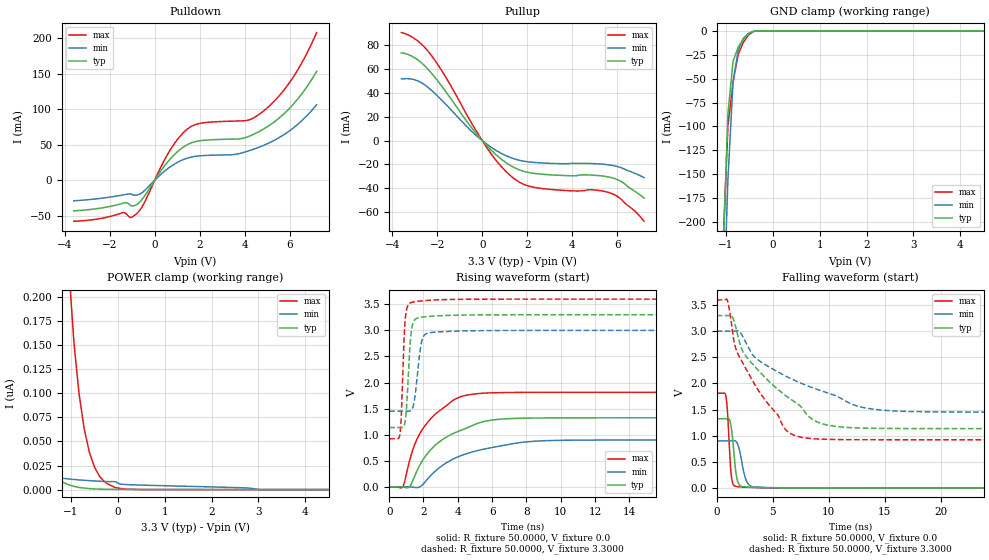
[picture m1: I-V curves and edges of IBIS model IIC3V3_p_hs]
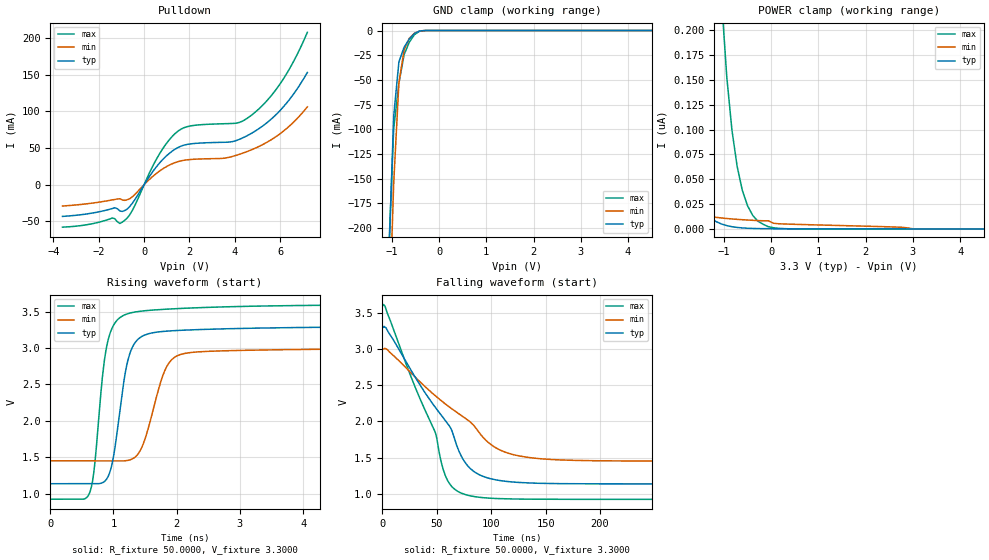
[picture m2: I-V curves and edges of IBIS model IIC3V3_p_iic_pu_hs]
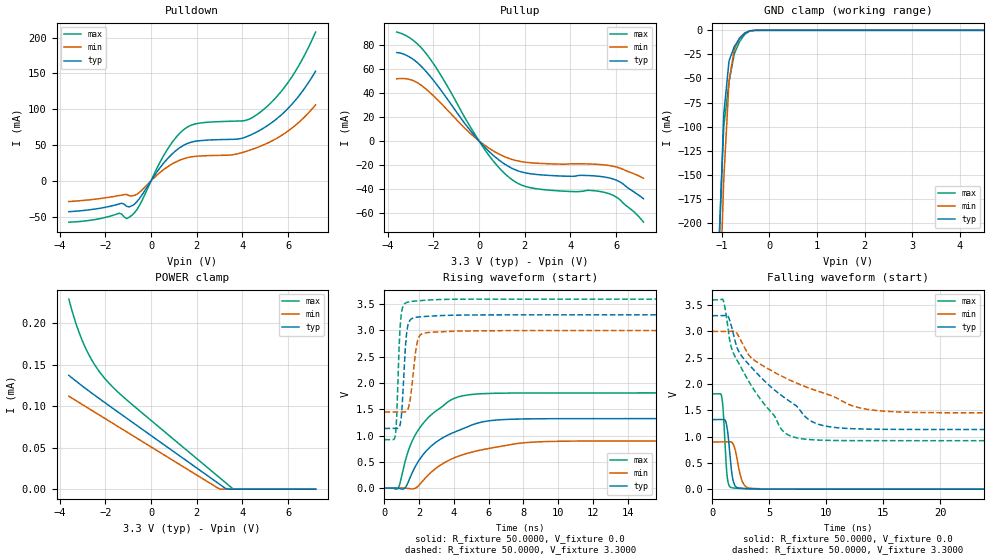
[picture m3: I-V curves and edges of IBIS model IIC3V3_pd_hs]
| IBIS file qfp64afe_3p3v.ibs generated by Viper version: 2020.12.17
[IBIS Ver]   5.0
[Comment Char]   |_char
[File Name]   qfp64afe_3p3v.ibs
[File Rev]   1.3
[Date]   Thu Dec 17 17:52:32 2020
[Source]   NXP Viper 2020.12.17
[Notes]
[Disclaimer] IMPORTANT NOTICE
  This information is provided on an AS IS basis and without warranty.
  IN NO EVENT SHALL NXP BE LIABLE FOR INCIDENTAL OR CONSEQUENTIAL
  DAMAGES ARISING FROM USE OF THIS INFORMATION. THIS DISCLAIMER OF
  WARRANTY EXTENDS TO THE USER OF THE INFORMATION, AND TO THEIR CUSTOMERS
  OR USERS OF PRODUCTS  AND IS IN LIEU OF ALL WARRANTIES WHETHER EXPRESS,
  IMPLIED, OR STATUTORY, INCLUDING IMPLIED WARRANTIES OF MERCHANTABILITY
  OR FITNESS FOR PARTICULAR PURPOSE.
  NXP does not represent or warrant that the information furnished
  hereunder is free of infringement of any third party patents,
  copyrights, trade secrets, or other intellectual property rights.
  NXP does not represent or warrant that the information is free of
  defect, or that it meets any particular standard, requirements or need
  of the user of the infomation or their customers.
  NXP reserves the right to change the information in this file
  without notice.
   http://www.nxp.com
[Copyright]   (C) Copyright NXP 2004 - 2020, All Rights Reserved.
|   qfp64Afe
[Component]   qfp64Afe
[Manufacturer]   NXP
[Package]
| variable   typ   min   max
R_pkg   0.18002   0.098036   0.22836
L_pkg   3.270e-09   2.478e-09   3.882e-09
C_pkg   4.877e-13   4.194e-13   6.388e-13
[Pin] signal_name   model_name   R_pin   L_pin   C_pin
1   P2_1   gpio   0.20176   3.768e-09 4.934e-13
2   OPAMP2_INN   NC   0.18655   3.432e-09 5.614e-13
3   P0_1   gpio   0.1882   3.425e-09 5.543e-13
4   P1_0   gpio   0.18167   3.391e-09 4.852e-13
5   ADC1IN1B   NC   0.17508   3.272e-09 4.734e-13
6   ADC1IN1A   NC   0.17211   3.184e-09 4.709e-13
7   P0_11   gpio   0.17322   3.095e-09 4.516e-13
8   VDDA   POWER   NA   NA   NA
9   VREF_OUT   NC   0.098933  2.478e-09 5.107e-13
10   VREFP   NC   0.098036  2.682e-09 4.989e-13
11   VREFN   NC   0.10339   2.593e-09 5.200e-13
12   VSSA   GND   NA   NA   NA
13   P0_16   gpio   0.18219   3.272e-09 4.683e-13
14   P0_10   gpio   0.18473   3.372e-09 4.943e-13
15   P0_15   gpio   0.1948   3.518e-09 5.647e-13
16   P0_31   gpio   0.21166   3.882e-09 5.047e-13
17   P0_8   gpio   0.19981   3.690e-09 4.818e-13
18   OPAMP0_INN   NC   0.18485   3.354e-09 5.404e-13
19   P0_27   gpio   0.1771   3.251e-09 5.158e-13
20   OPAMP1_INN   NC   0.17264   3.242e-09 4.518e-13
21   XTAL32M_N   NC   0.17308   3.207e-09 4.514e-13
22   XTAL32M_P   NC   0.17099   3.143e-09 4.435e-13
23   RESETN   gpio   0.17312   3.058e-09 4.290e-13
24   VDD_CORE   POWER   NA   NA   NA
25   P1_22   gpio   0.17347   2.976e-09 4.359e-13
26   P0_17   gpio   0.17222   3.063e-09 4.368e-13
27   P0_7   gpio   0.17974   2.960e-09 4.541e-13
28   VDDE_2   POWER   NA   NA   NA
29   VSS_MAIN_PWR   GND   NA   NA   NA
30   VSS_MAIN   GND   NA   NA   NA
31   LX   NC   0.12471   2.527e-09 6.388e-13
32   VDD_MAIN_PWR   NC   NA   NA   NA
33   XTAL32K_P   NC   0.20305   3.722e-09 4.831e-13
34   XTAL32K_N   NC   0.18797   3.388e-09 5.425e-13
35   VBAT   NC   0.17937   3.272e-09 4.763e-13
36   P0_0   gpio   0.17575   3.216e-09 4.542e-13
37   P0_9   gpio   0.17142   3.151e-09 4.522e-13
38   P0_18   gpio   0.17027   3.108e-09 4.408e-13
39   P1_13   gpio   0.17092   3.083e-09 4.194e-13
40   P1_1   gpio   0.17351   3.079e-09 4.367e-13
41   P0_26   gpio   0.17937   3.140e-09 4.480e-13
42   P1_2   gpio   0.18924   3.260e-09 4.417e-13
43   P1_3   gpio   0.20575   3.278e-09 4.623e-13
44   VDDE_4   POWER   NA   NA   NA
45   P0_24   gpio   0.18768   3.277e-09 4.591e-13
46   P0_13   iic   0.19613   3.445e-09 5.506e-13
47   P0_14   iic   0.20782   3.616e-09 5.657e-13
48   P0_20   gpio   0.21594   3.876e-09 4.850e-13
49   P0_21   gpio   0.20723   3.837e-09 4.904e-13
50   P0_22   gpio   0.1962   3.547e-09 5.661e-13
51   P0_25   gpio   0.18792   3.420e-09 5.062e-13
52   P0_2   gpio   0.18663   3.397e-09 4.750e-13
53   P1_15   gpio   0.17882   3.273e-09 4.700e-13
54   P0_19   gpio   0.17446   3.156e-09 4.633e-13
55   P0_3   gpio   0.17673   3.008e-09 4.457e-13
56   VDDE_4   POWER   NA   NA   NA
57   P0_4   gpio   0.17637   3.003e-09 4.457e-13
58   P1_16   gpio   0.17537   3.170e-09 4.476e-13
59   P0_6   gpio   0.17935   3.248e-09 4.687e-13
60   P0_5   gpio   0.18758   3.378e-09 4.757e-13
61   P0_29   gpio   0.19171   3.430e-09 4.834e-13
62   P1_11   gpio   0.20582   3.539e-09 5.647e-13
63   P0_30   gpio   0.22836   3.428e-09 5.818e-13
64   VDDE_4   POWER   NA   NA   NA
65   VSS   GND   NA   NA   NA
[Pin Mapping]   pulldown_ref   pullup_ref
1   VSS   VDDA
2   NC   NC
3   VSS   VDDA
4   VSS   VDDA
5   NC   NC
6   NC   NC
7   VSS   VDDA
8   NC   VDDA
9   NC   NC
10   NC   NC
11   NC   NC
12   VSSA   NC
13   VSS   VDDA
14   VSS   VDDA
15   VSS   VDDA
16   VSS   VDDA
17   VSS   VDDA
18   NC   NC
19   VSS   VDDA
20   NC   NC
21   NC   NC
22   NC   NC
23   VSS   VDDE_2
24   NC   VDD_CORE
25   VSS   VDDE_2
26   VSS   VDDE_2
27   VSS   VDDE_2
28   NC   VDDE_2
29   VSS_MAIN_PWR   NC
30   VSS_MAIN   NC
31   NC   NC
32   NC   NC
33   NC   NC
34   NC   NC
35   NC   NC
36   VSS   VDDE_4
37   VSS   VDDE_4
38   VSS   VDDE_4
39   VSS   VDDE_4
40   VSS   VDDE_4
41   VSS   VDDE_4
42   VSS   VDDE_4
43   VSS   VDDE_4
44   NC   VDDE_4
45   VSS   VDDE_4
46   VSS   VDDE_4
47   VSS   VDDE_4
48   VSS   VDDE_4
49   VSS   VDDE_4
50   VSS   VDDE_4
51   VSS   VDDE_4
52   VSS   VDDE_4
53   VSS   VDDE_4
54   VSS   VDDE_4
55   VSS   VDDE_4
56   NC   VDDE_4
57   VSS   VDDE_4
58   VSS   VDDE_4
59   VSS   VDDE_4
60   VSS   VDDE_4
61   VSS   VDDE_4
62   VSS   VDDE_4
63   VSS   VDDE_4
64   NC   VDDE_4
65   VSS   NC
|*   Model Selector   *
[Model Selector] gpio
MFIO3V3_pd_hs   EPUN=1 EPD=1 EHS=1
MFIO3V3_pd_ls   EPUN=1 EPD=1 EHS=0
MFIO3V3_pu_hs   EPUN=0 EPD=0 EHS=1
MFIO3V3_pu_ls   EPUN=0 EPD=0 EHS=0
MFIO3V3_p_hs   EPUN=1 EPD=0 EHS=1
MFIO3V3_p_ls   EPUN=1 EPD=0 EHS=0
MFIO3V3_r_hs   EPUN=0 EPD=1 EHS=1
MFIO3V3_r_ls   EPUN=0 EPD=1 EHS=0
[Model Selector] iic
IIC3V3_pd_hs   EGP=1 EPUN=1 EPD=1 EHS=1
IIC3V3_pd_ls   EGP=1 EPUN=1 EPD=1 EHS=0
IIC3V3_p_hs   EGP=1 EPUN=1 EPD=0 EHS=1
IIC3V3_p_ls   EGP=1 EPUN=1 EPD=0 EHS=0
IIC3V3_pu_hs   EGP=1 EPUN=0 EPD=0 EHS=1
IIC3V3_pu_ls   EGP=1 EPUN=0 EPD=0 EHS=0
IIC3V3_r_hs   EGP=1 EPUN=0 EPD=1 EHS=1
IIC3V3_r_ls   EGP=1 EPUN=0 EPD=1 EHS=0
IIC3V3_pd_iic_hs   EGP=0 ECS=0 EPUN=1 EPD=1
IIC3V3_p_iic_hs   EGP=0 ECS=0 EPUN=1 EPD=0
IIC3V3_pu_iic_hs   EGP=0 ECS=0 EPUN=0 EPD=0
IIC3V3_r_iic_hs   EGP=0 ECS=0 EPUN=0 EPD=1
IIC3V3_pd_iic_pu_hs   EGP=0 ECS=1 EPUN=1 EPD=1 SSEL=1
IIC3V3_p_iic_pu_hs   EGP=0 ECS=1 EPUN=1 EPD=0 SSEL=1
IIC3V3_pu_iic_pu_hs   EGP=0 ECS=1 EPUN=0 EPD=0 SSEL=1
IIC3V3_r_iic_pu_hs   EGP=0 ECS=1 EPUN=0 EPD=1 SSEL=1
| End [Component] qfp64Afe
| Models and submodels in the file (24): IIC3V3_p_hs (I/O), IIC3V3_p_iic_hs (I/O_open_drain), IIC3V3_p_iic_pu_hs (I/O_open_drain), IIC3V3_p_ls (I/O), IIC3V3_pd_hs (I/O), IIC3V3_pd_iic_hs (I/O_open_drain), IIC3V3_pd_iic_pu_hs (I/O_open_drain), IIC3V3_pd_ls (I/O), IIC3V3_pu_hs (I/O), IIC3V3_pu_iic_hs (I/O_open_drain), IIC3V3_pu_iic_pu_hs (I/O_open_drain), IIC3V3_pu_ls (I/O), IIC3V3_r_hs (I/O), IIC3V3_r_iic_hs (I/O_open_drain), IIC3V3_r_iic_pu_hs (I/O_open_drain), IIC3V3_r_ls (I/O), MFIO3V3_p_hs (I/O), MFIO3V3_p_ls (I/O), MFIO3V3_pd_hs (I/O), MFIO3V3_pd_ls (I/O), MFIO3V3_pu_hs (I/O), MFIO3V3_pu_ls (I/O), MFIO3V3_r_hs (I/O), MFIO3V3_r_ls (I/O)
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[Model] IIC3V3_p_hs
|   Model IIC3V3_p_hs
| This model was characterised for following simulation conditions:
| External (pad) voltage:
|   - Typ: 3.3V,   - Min: 3.0V,   - Max: 3.6V
| Library cells for typ/min/max conditions are connected as defined below:
|  IO - External Pad
|  A - Core Input
|  EN - Output Buffer Enable
|  BOOST - vdde
|  EGP - vdd
|  EHS - vdd
|  ENZI - vdd
|  EPD - gnd
|  EPUN - vdd
|  ZI - NC
|  ZIF - NC
|  gnd - gnd
|  gnde - gnde
|  vdd - vdd
|  vdde - vdde
| All other pins connected to ground
Model_type I/O
Polarity   Non-Inverting
Enable   Active-Low
Vinl =   0.9900V
Vinh =   2.3100V
Vmeas =  1.6500V
Cref =   0.0F
Rref =   1.0000k
Vref =   0.0V
C_comp   3.6227pF   3.4779pF   3.7656pF
|C_comp_pullup   0.9287pF   0.9115pF   0.9356pF
|C_comp_pulldown   2.3426pF   2.4945pF   2.1982pF
[Model Spec]
| variable   typ   min   max
Vinh   0.9900V   0.9000V   1.0800V
Vinl   2.3100V   2.1000V   2.5200V
Vmeas   1.6500V   1.5000V   1.8000V
[Temperature Range]   25.0000   0.1250k   -40.0000
[Voltage Range]   3.3000V   3.0000V   3.6000V
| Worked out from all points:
|   slope of the pulldown table from 0 to 0.495 V, typ, clamps not added: 22 ohm
|   slope of the pullup table from 0 to 0.495 V, typ, clamps not added: 50.2 ohm
|   GND clamp passes 1 mA (typ) near -0.43 V on its own axis
|   rising waveform, R_fixture 50.0000, V_fixture 0.0: 20-80 % time 2.42ns typ, 3.15ns min, 1.81ns max; typ from 0 V to 1.32 V
|   rising waveform, R_fixture 50.0000, V_fixture 3.3000: 20-80 % time 230ps typ, 322ps min, 186ps max; typ from 1.14 V to 3.3 V
|   falling waveform, R_fixture 50.0000, V_fixture 0.0: 20-80 % time 371ps typ, 535ps min, 282ps max; typ from 1.32 V to 0 V
|   falling waveform, R_fixture 50.0000, V_fixture 3.3000: 20-80 % time 5.52ns typ, 7.85ns min, 3.84ns max; typ from 3.3 V to 1.14 V
[Pulldown]
|Voltage   I(typ)   I(min)   I(max)
-3.6V     -43.22mA   -29.09mA   -57.9mA
-1.29V    -31.46mA   -20.15mA   -46.47mA
-1.07V    -35.79mA   -19.19mA   -52.9mA
-850mV    -35.14mA   -21.36mA   -48.43mA
-520mV    -25.35mA   -16.52mA   -35.11mA
580mV     25.81mA    16.3mA     36.8mA
1.24V     45.79mA    28.53mA    65.82mA
1.9V      54.89mA    33.9mA     79.08mA
4.1V      60.56mA    40.39mA    84.05mA
4.76V     70.46mA    47.89mA    95.34mA
6.08V     103.9mA    71.43mA    141.2mA
7.2V      153mA      106.1mA    207.7mA
[Pullup]
|Voltage   I(typ)   I(min)   I(max)
-3.6V     73.7mA     51.87mA    90.79mA
-2.92V    68.56mA    50.58mA    84.45mA
-2.26V    56.64mA    42.24mA    71.49mA
-1.6V     40.55mA    30.05mA    52.55mA
160mV     -3.402mA   -2.371mA   -4.704mA
820mV     -15.2mA    -10.46mA   -21.22mA
1.37V     -22.16mA   -15.02mA   -31.28mA
1.81V     -25.65mA   -17.18mA   -36.45mA
2.47V     -27.92mA   -18.56mA   -39.79mA
5.66V     -30.76mA   -20.47mA   -43.83mA
6.1V      -33.55mA   -22.29mA   -48.04mA
7.2V      -48.27mA   -31.2mA    -67.82mA
[GND_clamp]
|Voltage   I(typ)   I(min)   I(max)
-3.6V     -5.602A    -5.487A    -5.717A
-1.07V    -242mA     -316.8mA   -230.5mA
-960mV    -86.75mA   -154.7mA   -99.48mA
-850mV    -31.81mA   -53.08mA   -53.5mA
-740mV    -16.96mA   -19.87mA   -24.43mA
-630mV    -8.589mA   -7.919mA   -11.88mA
-520mV    -2.996mA   -2.727mA   -4.187mA
-410mV    -432.5uA   -495.8uA   -580.8uA
7.2V      0A         0A         0A
[POWER_clamp]
|Voltage   I(typ)   I(min)   I(max)
-3.6V     2.12uA     118.8nA    63.41uA
-3.03V    844.5nA    61.84nA    27.62uA
-2.37V    225.8nA    29.91nA    8.403uA
-2.04V    102.5nA    21.72nA    4.105uA
-1.82V    57.11nA    17.98nA    2.406uA
-1.49V    21.61nA    14.11nA    975.4nA
-1.05V    4.967nA    11.05nA    231.3nA
-830mV    2.261nA    10.06nA    99.54nA
-720mV    1.525nA    9.658nA    63.01nA
-500mV    718.9pA    8.985nA    23.37nA
-170mV    294.4pA    8.237nA    4.755nA
7.2V      0A         0A         0A
[Ramp]
| variable   typ   min   max
dV/dt_r  0.7941/2.4211n   0.5390/3.1525n   1.0875/1.8120n
dV/dt_f  1.2989/5.5187n   0.9297/7.8507n   1.6070/3.8381n
R_load = 50.0000
[Rising Waveform]
R_fixture= 50.0000
V_fixture= 0.0
V_fixture_min= 0.0
V_fixture_max= 0.0
|time   V(typ)   V(min)   V(max)
0s        2.243nV    52.63nV    27.54nV
783.4ps   -2.546mV   48.23uV    -3.663mV
1.2ns     6.371mV    -1.183mV   516.9mV
1.762ns   400.2mV    -5.572mV   1.005V
2.604ns   772.3mV    274.8mV    1.368V
3.633ns   1.006V     515.9mV    1.636V
5.446ns   1.245V     716.8mV    1.794V
7.589ns   1.314V     845.6mV    1.81V
17.45ns   1.323V     898mV      1.812V
1us       1.323V     898.3mV    1.813V
[Rising Waveform]
R_fixture= 50.0000
V_fixture= 3.3000
V_fixture_min= 3.0000
V_fixture_max= 3.6000
|time   V(typ)   V(min)   V(max)
0s        1.135V     1.45V      921.7mV
627.3ps   1.135V     1.45V      1.012V
700.7ps   1.134V     1.451V     1.326V
903.6ps   1.208V     1.45V      3.068V
1.101ns   2.057V     1.448V     3.484V
1.223ns   2.763V     1.454V     3.525V
1.356ns   3.105V     1.506V     3.542V
2.023ns   3.26V      2.9V       3.57V
4.301ns   3.294V     2.99V      3.597V
1us       3.3V       3V         3.6V
[Falling Waveform]
R_fixture= 50.0000
V_fixture= 0.0
V_fixture_min= 0.0
V_fixture_max= 0.0
|time   V(typ)   V(min)   V(max)
0s        1.323V     898.3mV    1.813V
822ps     1.323V     898.3mV    1.758V
972.4ps   1.326V     898.3mV    1.431V
1.252ns   1.222V     898.1mV    350.6mV
1.476ns   816.9mV    900.3mV    64.93mV
1.726ns   277.3mV    889.4mV    27.64mV
2.019ns   57.27mV    737.3mV    19.74mV
2.754ns   14.85mV    95.71mV    10.98mV
4.273ns   3.379mV    7.479mV    1.748mV
1us       13.95nV    73.04nV    34.74nV
[Falling Waveform]
R_fixture= 50.0000
V_fixture= 3.3000
V_fixture_min= 3.0000
V_fixture_max= 3.6000
|time   V(typ)   V(min)   V(max)
0s        3.3V       3V         3.6V
933.7ps   3.299V     3V         3.603V
1.389ns   3.287V     2.999V     3.037V
1.891ns   2.917V     3.01V      2.567V
2.697ns   2.498V     2.747V     2.246V
6.123ns   1.774V     2.146V     1.125V
10.95ns   1.17V      1.732V     925.1mV
14.46ns   1.14V      1.495V     922mV
24.74ns   1.135V     1.451V     921.7mV
1us       1.135V     1.45V      921.7mV
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[Model] IIC3V3_p_iic_pu_hs
|   Model IIC3V3_p_iic_pu_hs
| This model was characterised for following simulation conditions:
| External (pad) voltage:
|   - Typ: 3.3V,   - Min: 3.0V,   - Max: 3.6V
| Library cells for typ/min/max conditions are connected as defined below:
|  IO - External Pad
|  A - Core Input
|  EN - Output Buffer Enable
|  BOOST - vdde
|  ECS - vdd
|  EGP - gnd
|  ENZI - vdd
|  EPD - gnd
|  EPUN - vdd
|  SSEL - vdd
|  ZI - NC
|  ZIF - NC
|  gnd - gnd
|  gnde - gnde
|  vdd - vdd
|  vdde - vdde
| All other pins connected to ground
Model_type I/O_open_drain
Polarity   Non-Inverting
Enable   Active-Low
Vinl =   0.9900V
Vinh =   2.3100V
Vmeas =  1.6500V
Cref =   0.0F
Rref =   1.0000k
Vref =   3.3000V
C_comp   3.6227pF   3.4779pF   3.7656pF
|C_comp_pullup   0.9287pF   0.9114pF   0.9356pF
|C_comp_pulldown   2.3426pF   2.4946pF   2.1982pF
[Model Spec]
| variable   typ   min   max
Vinh   0.9900V   0.9000V   1.0800V
Vinl   2.3100V   2.1000V   2.5200V
Vmeas   1.6500V   1.5000V   1.8000V
Vref   3.3000V   3.0000V   3.6000V
Cref   0.0F   0.0F   0.0F
Rref   1.0000k   1.0000k   1.0000k
[Temperature Range]   25.0000   0.1250k   -40.0000
[Voltage Range]   3.3000V   3.0000V   3.6000V
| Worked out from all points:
|   slope of the pulldown table from 0 to 0.495 V, typ, clamps not added: 22 ohm
|   GND clamp passes 1 mA (typ) near -0.43 V on its own axis
|   rising waveform, R_fixture 50.0000, V_fixture 3.3000: 20-80 % time 227ps typ, 309ps min, 192ps max; typ from 1.14 V to 3.3 V
|   falling waveform, R_fixture 50.0000, V_fixture 3.3000: 20-80 % time 50.8ns typ, 68.7ns min, 38.5ns max; typ from 3.3 V to 1.14 V
[Pulldown]
|Voltage   I(typ)   I(min)   I(max)
-3.6V     -43.22mA   -29.09mA   -57.9mA
-1.29V    -31.46mA   -20.15mA   -46.47mA
-1.07V    -35.79mA   -19.19mA   -52.9mA
-850mV    -35.14mA   -21.36mA   -48.43mA
-520mV    -25.35mA   -16.52mA   -35.11mA
580mV     25.81mA    16.3mA     36.8mA
1.24V     45.79mA    28.53mA    65.82mA
1.9V      54.89mA    33.9mA     79.08mA
4.1V      60.56mA    40.39mA    84.05mA
4.76V     70.46mA    47.89mA    95.34mA
6.08V     103.9mA    71.43mA    141.2mA
7.2V      153mA      106.1mA    207.7mA
[GND_clamp]
|Voltage   I(typ)   I(min)   I(max)
-3.6V     -5.602A    -5.487A    -5.717A
-1.07V    -242mA     -316.8mA   -230.5mA
-960mV    -86.75mA   -154.7mA   -99.48mA
-850mV    -31.81mA   -53.08mA   -53.5mA
-740mV    -16.96mA   -19.87mA   -24.43mA
-630mV    -8.589mA   -7.919mA   -11.88mA
-520mV    -2.996mA   -2.727mA   -4.187mA
-410mV    -432.5uA   -495.8uA   -580.8uA
7.2V      0A         0A         0A
[POWER_clamp]
|Voltage   I(typ)   I(min)   I(max)
-3.6V     2.12uA     118.8nA    63.41uA
-3.03V    844.5nA    61.84nA    27.62uA
-2.37V    225.8nA    29.91nA    8.403uA
-2.04V    102.5nA    21.72nA    4.105uA
-1.82V    57.11nA    17.98nA    2.406uA
-1.49V    21.61nA    14.11nA    975.4nA
-1.05V    4.967nA    11.05nA    231.3nA
-830mV    2.261nA    10.06nA    99.54nA
-720mV    1.525nA    9.658nA    63.01nA
-500mV    718.9pA    8.985nA    23.37nA
-170mV    294.4pA    8.237nA    4.755nA
7.2V      0A         0A         0A
[Ramp]
| variable   typ   min   max
dV/dt_r  1.2989/0.2271n   0.9297/0.3090n   1.6070/0.1925n
dV/dt_f  1.2989/50.7796n   0.9297/68.6526n   1.6070/38.5019n
R_load = 50.0000
[Rising Waveform]
R_fixture= 50.0000
V_fixture= 3.3000
V_fixture_min= 3.0000
V_fixture_max= 3.6000
|time   V(typ)   V(min)   V(max)
0s        1.135V     1.45V      921.7mV
623.4ps   1.135V     1.45V      1.013V
886ps     1.193V     1.45V      2.995V
994ps     1.479V     1.45V      3.305V
1.153ns   2.48V      1.449V     3.448V
1.388ns   3.122V     1.544V     3.503V
1.807ns   3.231V     2.682V     3.534V
2.03ns    3.244V     2.903V     3.544V
5.603ns   3.294V     2.992V     3.595V
1us       3.3V       3V         3.6V
[Falling Waveform]
R_fixture= 50.0000
V_fixture= 3.3000
V_fixture_min= 3.0000
V_fixture_max= 3.6000
|time   V(typ)   V(min)   V(max)
0s        3.3V       3V         3.6V
2.46ns    3.303V     3.01V      3.593V
48.38ns   2.199V     2.358V     1.857V
54.58ns   2.076V     2.28V      1.407V
59.71ns   1.976V     2.22V      1.188V
72.76ns   1.512V     2.08V      1.006V
83.18ns   1.317V     1.957V     962.6mV
112.4ns   1.172V     1.577V     928.9mV
163.4ns   1.139V     1.467V     922.1mV
1us       1.135V     1.45V      921.7mV
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[Model] IIC3V3_pd_hs
|   Model IIC3V3_pd_hs
| This model was characterised for following simulation conditions:
| External (pad) voltage:
|   - Typ: 3.3V,   - Min: 3.0V,   - Max: 3.6V
| Library cells for typ/min/max conditions are connected as defined below:
|  IO - External Pad
|  A - Core Input
|  EN - Output Buffer Enable
|  BOOST - vdde
|  EGP - vdd
|  EHS - vdd
|  ENZI - vdd
|  EPD - vdd
|  EPUN - vdd
|  ZI - NC
|  ZIF - NC
|  gnd - gnd
|  gnde - gnde
|  vdd - vdd
|  vdde - vdde
| All other pins connected to ground
Model_type I/O
Polarity   Non-Inverting
Enable   Active-Low
Vinl =   0.9900V
Vinh =   2.3100V
Vmeas =  1.6500V
Cref =   0.0F
Rref =   1.0000k
Vref =   0.0V
C_comp   3.5907pF   3.4406pF   3.7387pF
|C_comp_pullup   0.9138pF   0.9000pF   0.9174pF
|C_comp_pulldown   2.3267pF   2.4802pF   2.1806pF
[Model Spec]
| variable   typ   min   max
Vinh   0.9900V   0.9000V   1.0800V
Vinl   2.3100V   2.1000V   2.5200V
Vmeas   1.6500V   1.5000V   1.8000V
[Temperature Range]   25.0000   0.1250k   -40.0000
[Voltage Range]   3.3000V   3.0000V   3.6000V
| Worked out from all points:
|   slope of the pulldown table from 0 to 0.495 V, typ, clamps not added: 22 ohm
|   slope of the pullup table from 0 to 0.495 V, typ, clamps not added: 50.2 ohm
|   GND clamp passes 1 mA (typ) near -0.43 V on its own axis
|   rising waveform, R_fixture 50.0000, V_fixture 0.0: 20-80 % time 2.41ns typ, 3.15ns min, 1.81ns max; typ from 0 V to 1.32 V
|   rising waveform, R_fixture 50.0000, V_fixture 3.3000: 20-80 % time 230ps typ, 322ps min, 186ps max; typ from 1.14 V to 3.3 V
|   falling waveform, R_fixture 50.0000, V_fixture 0.0: 20-80 % time 371ps typ, 533ps min, 281ps max; typ from 1.32 V to 0 V
|   falling waveform, R_fixture 50.0000, V_fixture 3.3000: 20-80 % time 5.51ns typ, 7.83ns min, 3.82ns max; typ from 3.3 V to 1.14 V
[Pulldown]
|Voltage   I(typ)   I(min)   I(max)
-3.6V     -43.22mA   -29.09mA   -57.9mA
-1.29V    -31.46mA   -20.15mA   -46.47mA
-1.07V    -35.79mA   -19.19mA   -52.9mA
-850mV    -35.14mA   -21.36mA   -48.43mA
-520mV    -25.35mA   -16.52mA   -35.11mA
580mV     25.81mA    16.3mA     36.8mA
1.24V     45.79mA    28.53mA    65.82mA
1.9V      54.89mA    33.9mA     79.08mA
4.1V      60.55mA    40.38mA    84.05mA
4.76V     70.44mA    47.87mA    95.32mA
6.08V     103.9mA    71.39mA    141.2mA
7.2V      152.9mA    106mA      207.6mA
[Pullup]
|Voltage   I(typ)   I(min)   I(max)
-3.6V     73.65mA    51.83mA    90.73mA
-2.92V    68.52mA    50.55mA    84.41mA
-2.26V    56.61mA    42.22mA    71.46mA
-1.6V     40.53mA    30.04mA    52.53mA
160mV     -3.403mA   -2.371mA   -4.704mA
820mV     -15.2mA    -10.46mA   -21.22mA
1.37V     -22.16mA   -15.02mA   -31.28mA
1.81V     -25.65mA   -17.18mA   -36.45mA
2.47V     -27.92mA   -18.56mA   -39.79mA
5.66V     -30.76mA   -20.47mA   -43.83mA
6.1V      -33.55mA   -22.29mA   -48.04mA
7.2V      -48.27mA   -31.2mA    -67.82mA
[GND_clamp]
|Voltage   I(typ)   I(min)   I(max)
-3.6V     -5.602A    -5.487A    -5.717A
-1.07V    -242mA     -316.8mA   -230.5mA
-960mV    -86.76mA   -154.7mA   -99.49mA
-850mV    -31.82mA   -53.09mA   -53.51mA
-740mV    -16.97mA   -19.87mA   -24.44mA
-630mV    -8.597mA   -7.926mA   -11.89mA
-520mV    -3.004mA   -2.733mA   -4.196mA
-410mV    -439.7uA   -501.8uA   -589.4uA
7.2V      0A         0A         0A
[POWER_clamp]
|Voltage   I(typ)   I(min)   I(max)
-3.6V     137uA      111.9uA    228.9uA
-3.47V    134.1uA    109.7uA    215.6uA
-3.25V    129.3uA    106uA      196.2uA
-2.92V    122.3uA    100.4uA    172.9uA
-2.48V    113.3uA    92.88uA    150.2uA
-2.04V    104.5uA    85.42uA    133.7uA
-1.16V    87.2uA     70.51uA    109.7uA
2.91V     7.626uA    1.527uA    15.86uA
3.02V     5.475uA    0A         13.33uA
3.24V     1.173uA    0A         8.273uA
3.57V     0A         0A         687.1nA
7.2V      0A         0A         0A
[Ramp]
| variable   typ   min   max
dV/dt_r  0.7935/2.4144n   0.5386/3.1478n   1.0867/1.8089n
dV/dt_f  1.2983/5.5124n   0.9293/7.8350n   1.6062/3.8243n
R_load = 50.0000
[Rising Waveform]
R_fixture= 50.0000
V_fixture= 0.0
V_fixture_min= 0.0
V_fixture_max= 0.0
|time   V(typ)   V(min)   V(max)
0s        2.145nV    50.58nV    26.14nV
784.7ps   -2.611mV   49.1uV     -3.137mV
1.202ns   7.028mV    -1.221mV   519mV
1.771ns   405.7mV    -4.318mV   1.01V
2.618ns   776.7mV    279.1mV    1.373V
3.639ns   1.007V     517.2mV    1.637V
5.503ns   1.249V     720.8mV    1.794V
7.438ns   1.312V     838.3mV    1.809V
17.91ns   1.322V     897.4mV    1.811V
1us       1.322V     897.6mV    1.811V
[Rising Waveform]
R_fixture= 50.0000
V_fixture= 3.3000
V_fixture_min= 3.0000
V_fixture_max= 3.6000
|time   V(typ)   V(min)   V(max)
0s        1.135V     1.45V      921.3mV
628ps     1.134V     1.45V      1.013V
701.4ps   1.133V     1.45V      1.33V
904.8ps   1.209V     1.449V     3.073V
1.102ns   2.066V     1.447V     3.485V
1.223ns   2.761V     1.453V     3.525V
1.356ns   3.104V     1.505V     3.541V
2.025ns   3.259V     2.9V       3.569V
4.329ns   3.293V     2.989V     3.596V
1us       3.299V     2.999V     3.598V
[Falling Waveform]
R_fixture= 50.0000
V_fixture= 0.0
V_fixture_min= 0.0
V_fixture_max= 0.0
|time   V(typ)   V(min)   V(max)
0s        1.322V     897.6mV    1.811V
823ps     1.322V     897.6mV    1.756V
974.3ps   1.325V     897.6mV    1.423V
1.254ns   1.218V     897.5mV    343.4mV
1.479ns   809.6mV    899.6mV    62.93mV
1.72ns    284.1mV    889.7mV    27.16mV
2.013ns   58.28mV    741.7mV    19.25mV
2.763ns   14.33mV    92.17mV    10.48mV
4.222ns   3.365mV    7.6mV      1.686mV
1us       13.83nV    70.96nV    33.33nV
[Falling Waveform]
R_fixture= 50.0000
V_fixture= 3.3000
V_fixture_min= 3.0000
V_fixture_max= 3.6000
|time   V(typ)   V(min)   V(max)
0s        3.299V     2.999V     3.598V
922.2ps   3.298V     2.999V     3.606V
1.378ns   3.29V      2.998V     3.054V
1.853ns   2.949V     3.007V     2.582V
2.668ns   2.504V     2.757V     2.255V
6.08ns    1.779V     2.149V     1.135V
10.78ns   1.173V     1.748V     925.2mV
14.53ns   1.139V     1.493V     921.7mV
23.45ns   1.135V     1.451V     921.4mV
1us       1.135V     1.45V      921.3mV
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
